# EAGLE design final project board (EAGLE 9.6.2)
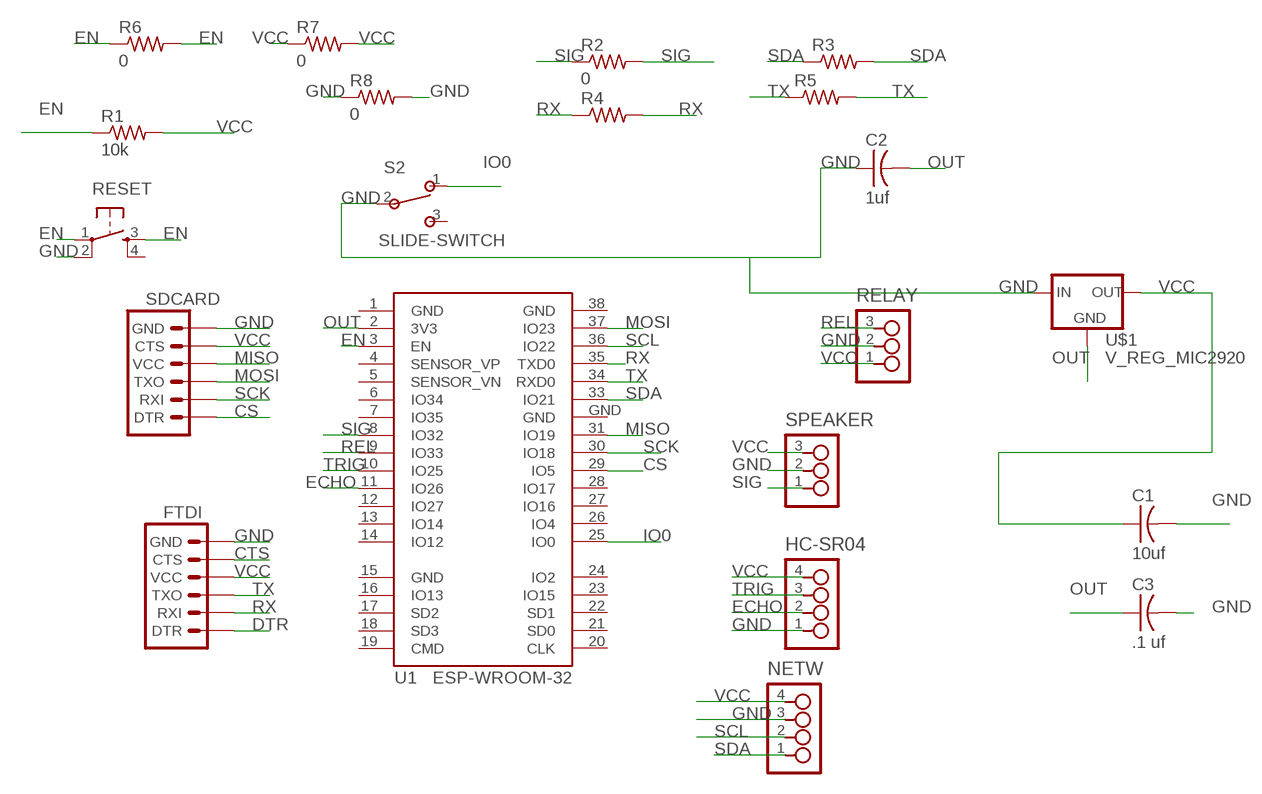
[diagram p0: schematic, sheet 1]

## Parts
C1  10uf  CAP-US1206  [C1206]
C2  1uf  CAP-US1206  [C1206]
C3  .1 uf  CAP-US1206  [C1206]
FTDI  FTDI_CONNECTORSMD  [1X06]
HC-SR04  4_PIN_HEADERHEADER  [SMT_PINS_4]
NETW  4_PIN_HEADERHEADER  [SMT_PINS_4]
R1  10k  RES-US1206  [R1206]
R2  0  RES-US1206  [R1206]
R3  RES-US1206  [R1206]
R4  RES-US1206  [R1206]
R5  RES-US1206  [R1206]
R6  0  RES-US1206  [R1206]
R7  0  RES-US1206  [R1206]
R8  0  RES-US1206  [R1206]
RELAY  3_PIN_HEADERHEADER  [SMT_PINS_3]
RESET  6MM_SWITCH6MM_SWITCH  [6MM_SWITCH]
S2  SLIDE-SWITCH  [AYZ0102AGRLC]
SDCARD  FTDI_CONNECTORSMD  [1X06]
SPEAKER  3_PIN_HEADERHEADER  [SMT_PINS_3]
U1  ESP-WROOM-32  [ESP-WROOM-32]
U$1  V_REG_MIC2920  [SOT223]

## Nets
CS: SDCARD.1(DTR) U1.29(IO5)
CTS: FTDI.5(CTS)
DTR: FTDI.1(DTR)
ECHO: HC-SR04.2 U1.11(IO26)
EN: R1.1 R6.1 R6.2 RESET.1(P) RESET.3(S) U1.3(EN)
GND: C1.2 C2.1 C3.2 FTDI.6(GND) HC-SR04.1 NETW.3 R8.1 R8.2 RELAY.2 RESET.2(P1) S2.2 SDCARD.6(GND) SPEAKER.2 U$1.1(IN)
IO0: S2.1 U1.25(IO0)
MISO: SDCARD.4(VCC) U1.31(IO19)
MOSI: SDCARD.3(TXO) U1.37(IO23)
OUT: C2.2 C3.1 U1.2(3V3) U$1.2(GND)
REL: RELAY.3 U1.9(IO33)
RX: FTDI.2(RXI) R4.1 R4.2 U1.35(TXD0)
SCK: SDCARD.2(RXI) U1.30(IO18)
SCL: NETW.2 U1.36(IO22)
SDA: NETW.1 R3.1 R3.2 U1.33(IO21)
SIG: R2.1 R2.2 SPEAKER.1 U1.8(IO32)
TRIG: HC-SR04.3 U1.10(IO25)
TX: FTDI.3(TXO) R5.1 R5.2 U1.34(RXD0)
VCC: C1.1 FTDI.4(VCC) HC-SR04.4 NETW.4 R1.2 R7.1 R7.2 RELAY.1 SDCARD.5(CTS) SPEAKER.3 U$1.3(OUT)
Unconnected: RESET.4(S1) S2.3 U1.4(SENSOR_VP) U1.5(SENSOR_VN) U1.6(IO34) U1.7(IO35) U1.12(IO27) U1.13(IO14) U1.14(IO12) U1.16(IO13) U1.17(SD2) U1.18(SD3) U1.19(CMD) U1.20(CLK) U1.21(SD0) U1.22(SD1) U1.23(IO15) U1.24(IO2) U1.26(IO4) U1.27(IO16) U1.28(IO17)

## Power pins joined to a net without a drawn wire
GND: U1.1(GND) U1.15(GND) U1.38(GND) U1.GND

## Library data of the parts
C1-C3 = fab:CAP-US
FTDI SDCARD = fablab:FTDI_CONNECTOR: FTDI connector smd
HC-SR04 NETW = fablab:4_PIN_HEADER: 4 SMT pin pads
R1-R8 = fab:RES-US: Resistor (US Symbol)
RELAY SPEAKER = fablab:3_PIN_HEADER: 3 SMT pin pads
RESET = fab:6MM_SWITCH: OMRON SWITCH
S2 = fab:SLIDE-SWITCH: SMD slide-switch AYZ0102AGRLC as found in the fablab inventory. Includes the mounting holes. Made by Zaerc.
U1 = esp32:ESP-WROOM-32: Espressif Systems ESP-WROOM-32
U$1 = fablab:V_REG_MIC2920: MIC2920A (http://www.micrel.com/_PDF/mic2920.pdf) - 400mA output LDO Regulator

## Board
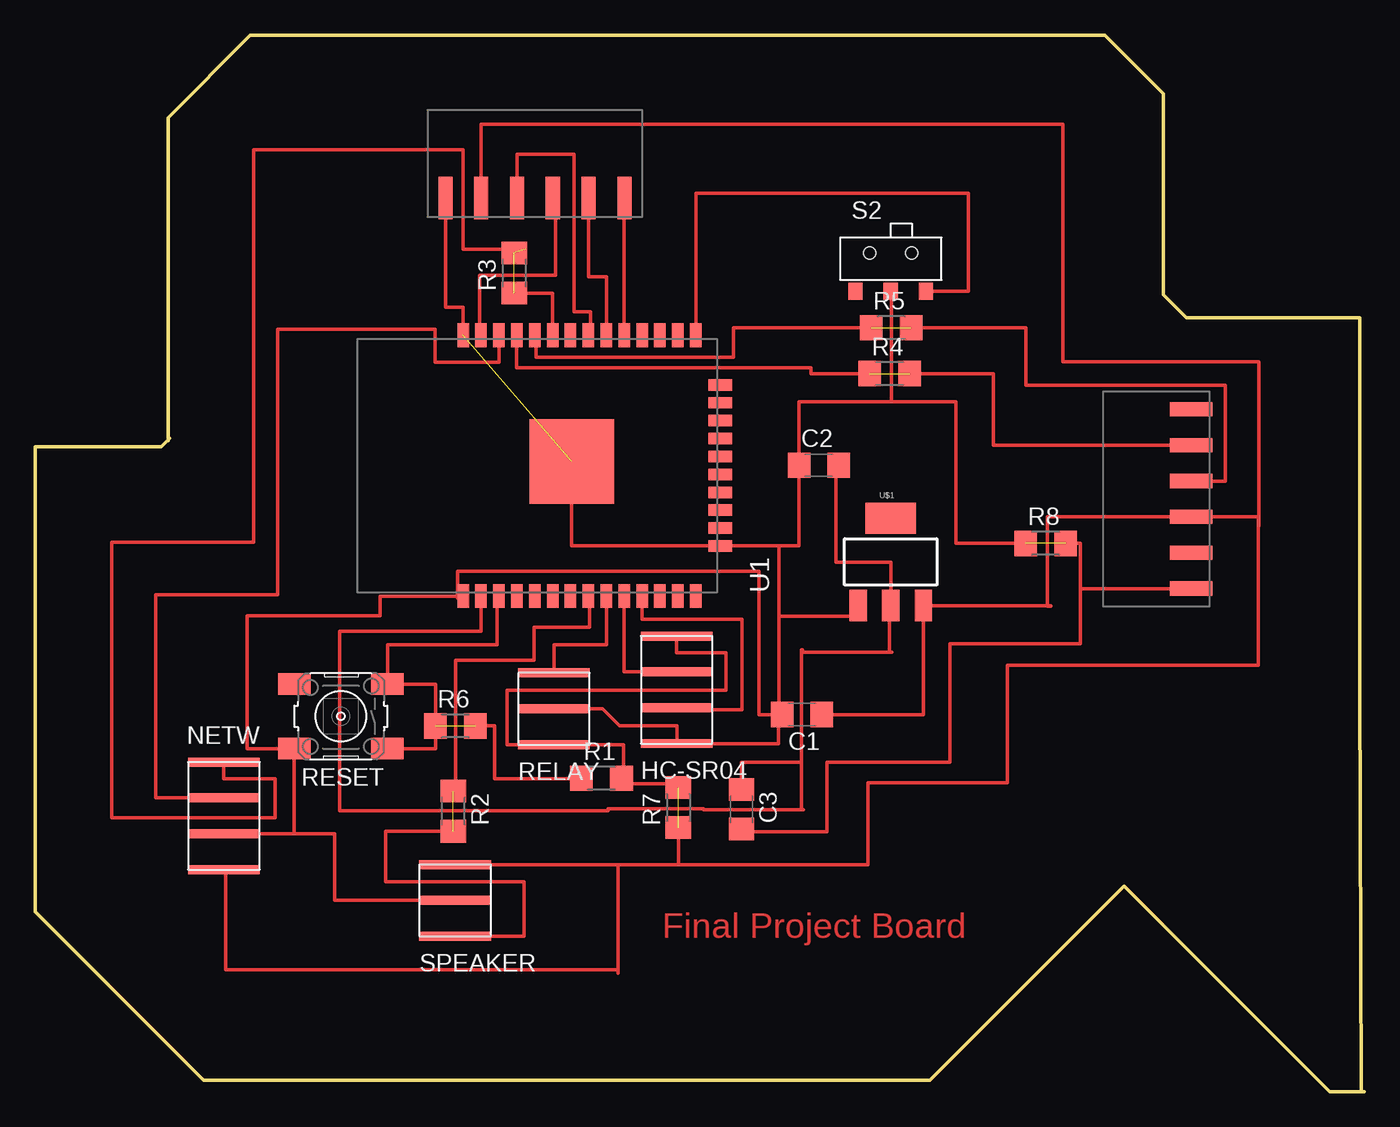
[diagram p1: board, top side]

Size 94.31 x 74.93 mm. Coordinates in mm from the lower left corner, seen from the top.
Outline: 9.42,46.18 9.42,69.09 15.27,74.93 75.89,74.93 80.06,70.76 80.06,56.52 81.69,54.89 94.01,54.89 94.01,29.06 94.08,0
Outline: 9.52,46.33 8.94,45.75 0,45.75 0,12.75 11.96,0.79 63.47,0.79 77.24,14.55
Outline: 77.29,14.55 91.85,0 94.31,0
Copper layers (1*16): Top 0.035mm / dielectric 1.5mm / Bottom 0.035mm
Design rules "default *": minimum track width 10mil, minimum drill 0.35mm, track to track 10mil, track to pad 10mil, pad to pad 10mil, via to via 10mil, smd to smd 6mil, copper to edge 40mil, drill to drill 6mil, minimum pad ring 10mil, minimum via ring 8mil, stop-mask expansion 4mil, vias tented up to drill 0mil, thermal gap 10mil

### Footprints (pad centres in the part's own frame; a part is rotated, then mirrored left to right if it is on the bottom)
C1206 = smd 1.6 x 1.8: 1 -1.4,0; 2 1.4,0
1X06 = smd 1 x 3: 1 -6.35,5; 2 -3.81,5; 3 -1.27,5; 4 1.27,5; 5 3.81,5; 6 6.35,5
SMT_PINS_4 = smd 5.08 x 0.635: 1 0,0; 2 0,2.54; 3 0,5.08; 4 0,7.62
R1206 = smd 1.6 x 1.803: 1 -1.422,0; 2 1.422,0
SMT_PINS_3 = smd 5.08 x 0.635: 1 0,0; 2 0,2.54; 3 0,5.08
6MM_SWITCH = smd 2.286 x 1.524: 1 -3.302,2.286; 2 3.302,2.286; 3 -3.302,-2.286; 4 3.302,-2.286
AYZ0102AGRLC = smd 1 x 1.2: 1 2.5,-2.3; 2 0,-2.3; 3 -2.5,-2.3 | hole 0.85: -1.5,0.4; 1.5,0.4
ESP-WROOM-32 = smd 1.676 x 0.813: 1 -9.25,7; 2 -9.25,5.73; 3 -9.25,4.46; 4 -9.25,3.19; 5 -9.25,1.92; 6 -9.25,0.65; 7 -9.25,-0.62; 8 -9.25,-1.89; 9 -9.25,-3.16; 10 -9.25,-4.43; 11 -9.25,-5.7; 12 -9.25,-6.97; 13 -9.25,-8.24; 14 -9.25,-9.51; 25 9.25,-9.51; 26 9.25,-8.24; 27 9.25,-6.97; 28 9.25,-5.7; 29 9.25,-4.43; 30 9.25,-3.16; 31 9.25,-1.89; 32 9.25,-0.62; 33 9.25,0.65; 34 9.25,1.92; 35 9.25,3.19; 36 9.25,4.46; 37 9.25,5.73; 38 9.25,7 | smd 0.813 x 1.676: 15 -5.7,-11.25; 16 -4.43,-11.25; 17 -3.16,-11.25; 18 -1.89,-11.25; 19 -0.62,-11.25; 20 0.65,-11.25; 21 1.92,-11.25; 22 3.19,-11.25; 23 4.46,-11.25; 24 5.73,-11.25 | smd 6 x 6: GND 0.3,-0.7
SOT223 = smd 1.219 x 2.235: 1 -2.311,-3.099; 2 0,-3.099; 3 2.311,-3.099 | smd 3.6 x 2.2: 4 0,3.099

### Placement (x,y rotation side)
C1  54.41,26.75 180 top
C2  55.6,44.42 0 top
C3  50.11,20.02 270 top
FTDI  77.01,42.04 270 top
HC-SR04  45.52,24.69 0 top
NETW  13.39,23.37 180 top
R1  40.18,22.23 0 top
R2  29.67,19.89 270 top
R3  33.99,58.06 90 top
R4  60.63,50.93 0 top
R5  60.73,54.18 0 top
R6  29.82,25.93 0 top
R7  45.64,20.14 90 top
R8  71.7,38.89 0 top
RELAY  36.8,24.61 0 top
RESET  21.69,26.62 180 top
S2  60.71,59.08 0 top
SDCARD  35.46,68.38 180 top
SPEAKER  29.79,11.02 0 top
U1  37.36,44.4 90 top
U$1  60.71,37.57 0 top

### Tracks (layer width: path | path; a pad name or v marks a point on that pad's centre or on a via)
CS
  Top 0.254: SDCARD.1 41.79,63.38 U1.29
ECHO
  Top 0.254: U1.11 43.06,33.5 50.14,33.5 50.14,27.08 45.52,27.08 HC-SR04.2
EN  (1 unrouted)
  Top 0.254: U1.3 32.78,35.02 32.78,31.7 24.99,31.7 RESET.3 28.4,28.91 R6.1 28.4,24.33 RESET.1 | R6.2 32.59,25.93 32.59,22.2 38.76,22.2 R1.1
GND  (2 unrouted)
  Top 0.254: 52.78,26.75 C1.2 51.36,26.75 51.36,36.91 29.97,36.91 29.97,35 30.36,35 U1.1 24.46,35.15 24.46,33.76 15.04,33.76 15.04,24.33 RESET.2 18.39,18.29 | 52.78,26.75 52.73,26.75 52.73,24.69 HC-SR04.1 45.54,24.69 45.54,25.96 41.45,25.96 40.26,27.15 RELAY.2 | 52.78,38.7 U1.15 38.06,38.7 U1.GND | 52.78,26.75 52.78,33.73 | 52.78,33.73 52.78,38.7 | FTDI.6 82.01,35.66 74.17,35.66 | 74.17,35.66 74.17,31.78 64.92,31.78 64.92,23.37 56.18,23.37 56.18,18.42 50.11,18.42 C3.2 | SDCARD.6 29.11,55.63 30.36,55.63 U1.38 | SPEAKER.2 21.26,13.56 21.26,18.29 18.39,18.29 | NETW.3 18.39,18.29 | 60.76,48.92 54.2,48.92 C2.1 54.2,38.7 52.78,38.7 | 60.76,48.92 60.76,56.78 S2.2 | U$1.1 58.39,33.73 52.78,33.73 | R8.2 74.17,38.89 74.17,35.66 | R8.1 65.33,38.89 65.33,48.92 60.76,48.92
IO0
  Top 0.254: S2.1 66.22,56.78 66.22,63.73 46.89,63.73 46.89,53.66 U1.25
MISO
  Top 0.254: SDCARD.4 34.19,66.47 38.23,66.47 38.23,55.32 39.42,55.32 39.42,53.65 U1.31
MOSI
  Top 0.254: SDCARD.3 36.93,63.17 36.93,57.91 31.52,57.91 31.52,53.65 U1.37
OUT
  Top 0.254: 31.43,34.95 U1.2 31.63,32.64 21.62,32.64 21.62,19.91 40.65,19.91 40.65,20.05 47.43,20.05 47.43,19.99 54.38,19.99 | 54.38,19.99 54.51,19.99 | 54.38,19.99 54.38,23.37 | 54.38,23.37 54.38,31.17 | 54.38,31.17 54.38,31.34 54.46,31.34 | 54.38,31.17 60.6,31.17 | 60.6,31.17 60.78,31.17 | 60.6,31.17 60.6,34.47 U$1.2 60.71,37.54 56.82,37.54 56.82,44.42 C2.2 | 54.38,23.37 50.11,23.37 C3.1 49.43,20.73
REL
  Top 0.254: RELAY.3 36.8,31.7 40.52,31.7 U1.9
RX  (1 unrouted)
  Top 0.254: FTDI.2 68,45.85 68,50.93 R4.2 | R4.1 55.04,50.93 55.04,51.33 34.16,51.33 34.16,53.65 U1.35
SCK
  Top 0.254: SDCARD.2 39.27,57.79 40.52,57.79 U1.30
SCL
  Top 0.254: NETW.2 8.53,20.83 8.53,35.26 17.2,35.26 17.2,54.08 28.37,54.08 28.37,51.74 28.55,51.74 32.9,51.74 U1.36
SDA  (2 unrouted)
  Top 0.254: NETW.1 13.39,22.17 17.02,22.17 17.02,19.41 5.44,19.41 5.44,38.96 15.49,38.96 15.49,66.8 30.35,66.8 30.35,59.77 34.8,59.77 | R3.1 36.71,56.64 U1.33
SIG  (1 unrouted)
  Top 0.254: SPEAKER.1 34.67,11.02 34.67,14.88 24.87,14.88 24.87,18.47 R2.2 | R2.2 | R2.1 29.84,21.49 29.84,30.58 35.38,30.58 35.38,32.92 39.32,32.92 39.32,35.15 U1.8
TRIG
  Top 0.254: U1.10 41.79,29.77 HC-SR04.3
TX  (1 unrouted)
  Top 0.254: FTDI.3 84.45,43.31 84.45,50.09 70.31,50.09 70.31,54.18 R5.2 | U1.34 35.53,53.65 35.53,52.09 49.56,52.09 49.56,54.18 R5.1
VCC  (1 unrouted)
  Top 0.254: RELAY.1 36.86,24.66 | C1.1 63.02,26.75 U$1.3 72.08,34.47 72.08,34.44 71.81,34.44 71.81,40.77 FTDI.4 86.79,40.77 86.79,40.11 | SPEAKER.3 59.08,16.1 59.08,21.92 68.99,21.92 68.99,30.25 86.79,30.25 86.79,40.11 | SPEAKER.3 41.35,16.1 41.35,8.64 | 41.35,8.64 41.35,8.38 | NETW.4 13.51,15.75 13.51,8.64 41.35,8.64 | SDCARD.5 31.65,68.63 72.92,68.63 72.92,51.77 86.82,51.77 86.82,40.11 86.79,40.11 | HC-SR04.4 45.52,31.14 49.02,31.14 49.02,28.47 33.49,28.47 33.49,24.61 RELAY.1 | R1.2 41.6,21.84 41.73,21.84 | 41.73,21.84 41.73,24.59 36.8,24.59 RELAY.1 | SPEAKER.3 45.64,16.1 R7.1 | R7.2 45.64,21.84 41.73,21.84

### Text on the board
Top: Final Project Board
